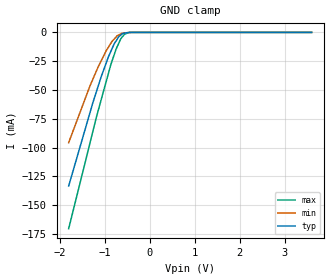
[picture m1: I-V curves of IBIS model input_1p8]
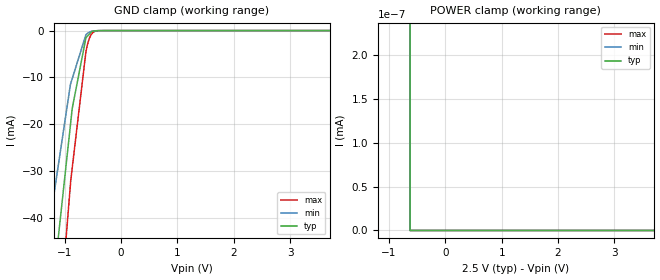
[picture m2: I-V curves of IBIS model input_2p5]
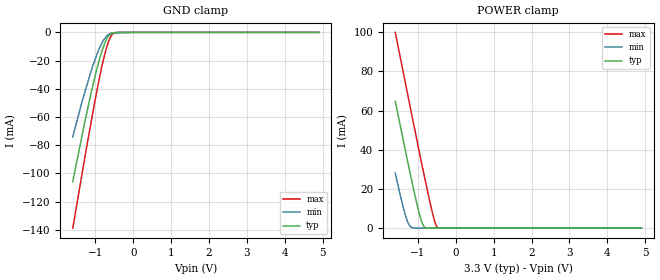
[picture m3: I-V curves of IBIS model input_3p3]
| Texas Instruments Incorporated
| 2N7001T-Q1 Single-Bit Dual-Supply Buffered Voltage Signal Converter
[IBIS Ver]   4.1
[File name]   2n7001t-q1.ibs
[File Rev]   1.0
[Date]   05/25/2018
[Source]
| Texas Instruments Incorporated.
| Analog-eLab Design Center, HPA
| 12500 TI Blvd
| Dallas, TX -75243
[Notes]   Revision History:
| Rev 1.0: 05/25/2018
| - Initial version of the model.
| - Model generated from simulations in SPECTRE.
| - C_comp although listed in numerical order of value are
|   obtained from varying PVT conditions. For PVT conditions for
|   each specific value refer the buffer description under
|   respective [Model]. IBIS model user is responsible for using
|   appropriate C_comp to simulate for Signal Integrity.
| - Model names with a trailing _1p8 contain the model for 1.8V operation.
|   Model names with a trailing _2p5 contain the model for 2.5V operation.
|   Model names with a trailing _3p3 contain the model for 3.3V operation.
[Disclaimer]
| This model is designed as an aid for customers of Texas Instruments.
| TI and its licensors and suppliers make no warranties, either expressed
| or implied, with respect to this  model, including the warranties of
| merchantability or fitness for a particular purpose. The model is
| provided solely on an "as is" basis. The entire risk as to its quality
| and performance is with the customer.
| This model is subject to change without notice. Texas Instruments
| Incorporated is not responsible for updating this model.
[Copyright]
(C) Copyright 2018 Texas Instruments Incorporated.All rights reserved.
|  Component 2N7001TQDCKRQ1 5-pin SC70 - DCK Package
|  Part # 2N7001TQDCKRQ1
[Component]   2N7001TQDCKRQ1
[Manufacturer]   TI
[Package]   |5 SC70 - DCK Package
|   typ   min   max
R_pkg   0.05   0.04   0.06
L_pkg   1.0nH   0.8nH   1.2nH
C_pkg   0.2pF   0.16pF   0.24pF
[Pin]   signal_name   model_name   R_pin   L_pin   C_pin
1   B   output   NA   NA   NA
2   VCCB   power   NA   NA   NA
3   GND   gnd   NA   NA   NA
4   A   input   NA   NA   NA
5   VCCA   power   NA   NA   NA
|   Model Selectors
[Model Selector]   output
output_1p8   1.8V   Digital Output
output_2p5   2.5V   Digital Output
output_3p3   3.3V   Digital Output
[Model Selector]   input
input_1p8   1.8V   Digital Input
input_2p5   2.5V   Digital Input
input_3p3   3.3V   Digital Input
| Models and submodels in the file (6): input_1p8 (Input), input_2p5 (Input), input_3p3 (Input), output_1p8 (Output), output_2p5 (Output), output_3p3 (Output)
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|   input_1p8 Model
[Model]   input_1p8
Model_type   Input
Vinl = 0.63
Vinh = 1.17
|   typ   min   max
C_comp   0.4871pF   0.3678pF   0.7475pF
|  Where Nom  PVT is Nominal Process,   1.8V,  27C
|   Fast PVT is Strong Process,   1.95V, -40C
|   Slow PVT is Weak Process,   1.65V, 130C
[Model spec]
|subparameter
Vinl   0.63   0.578   0.683
Vinh   1.17   1.073   1.268
[Voltage Range]   1.8   1.65   1.95
|Junction Temperature
[Temperature Range]   27   130   -40
[Power Clamp Reference]   1.8   1.65   1.95
[GND Clamp Reference]   0   0   0
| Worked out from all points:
|   GND clamp passes 1 mA (typ) near -0.60 V on its own axis
[GND Clamp]
|   Voltage   I(typ)   I(min)   I(max)
-1.8V     -133.4mA   -95.76mA   -170.5mA
-1.329V   -70.02mA   -46.69mA   -96.49mA
-1.176V   -50.62mA   -32.84mA   -72.54mA
-1.076V   -38.35mA   -24.46mA   -58.21mA
-918.3mV  -21.41mA   -12.94mA   -35.86mA
-862mV    -16.42mA   -9.398mA   -27.85mA
-743.7mV  -7.233mA   -3.863mA   -14.32mA
-686.9mV  -3.715mA   -2.245mA   -9.459mA
-640.9mV  -2.343mA   -1.317mA   -5.512mA
-555.4mV  -622.7uA   -479.8uA   -1.411mA
-372.2mV  -3.465uA   -6.978uA   -8.321uA
3.6V      0A         0A         0A
[POWER Clamp]
|   Voltage   I(typ)   I(min)   I(max)
-1.8V     0A         0A         0A
0V        0A         0A         0A
3.6V      0A         0A         0A
|   input_2p5 Model
[Model]   input_2p5
Model_type   Input
Vinl = 0.7
Vinh = 1.6
|   typ   min   max
C_comp   0.6021pF   0.407pF   0.8544pF
|  Where Nom  PVT is Nominal Process,   2.5V,  27C
|   Fast PVT is Strong Process,   2.7V, -40C
|   Slow PVT is Weak Process,   2.3V, 130C
[Voltage Range]   2.5   2.3   2.7
|Junction Temperature
[Temperature Range]   27   130   -40
[Power Clamp Reference]   2.5   2.3   2.7
[GND Clamp Reference]   0   0   0
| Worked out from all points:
|   GND clamp passes 1 mA (typ) near -0.58 V on its own axis
|   POWER clamp passes 1 mA (typ) near -1.65 V on its own axis
[GND Clamp]
|   Voltage   I(typ)   I(min)   I(max)
-2.5V     -235.9mA   -175.5mA   -1.819A
-1.353V   -73.9mA    -50.2mA    -99.92mA
-1.273V   -62.98mA   -41.43mA   -88.06mA
-1.222V   -56.03mA   -37.34mA   -80.51mA
-899.7mV  -20.15mA   -11.48mA   -32.82mA
-868.2mV  -16.64mA   -10.27mA   -29.34mA
-625mV    -1.529mA   -877.6uA   -4.494mA
-583.8mV  -1.011mA   -466.9uA   -2.4mA
-560.4mV  -718uA     -339.6uA   -1.561mA
-514.7mV  -165.9uA   -140.6uA   -575.4uA
-409.2mV  -13.07uA   -21.38uA   -29.47uA
5V        0A         0A         0A
[POWER Clamp]
|   Voltage   I(typ)   I(min)   I(max)
-2.5V     74.25mA    46.22mA    99.87mA
-1.342V   32.99uA    19.24uA    58.86uA
-625mV    0A         175pA      120.1pA
-624.9mV  0A         135.8pA    0A
-624.9mV  0A         0A         0A
5V        0A         0A         0A
|   input_3p3 Model
[Model]   input_3p3
Model_type   Input
Vinl = 0.8
Vinh = 2.0
|   typ   min   max
C_comp   0.6977pF   0.4525pF   0.8988pF
|  Where Nom  PVT is Nominal Process,   3.3V,  27C
|   Fast PVT is Strong Process,   3.6V, -40C
|   Slow PVT is Weak Process,   3V, 130C
[Voltage Range]   3.3   3   3.6
|Junction Temperature
[Temperature Range]   27   130   -40
[Power Clamp Reference]   3.3   3   3.6
[GND Clamp Reference]   0   0   0
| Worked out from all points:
|   GND clamp passes 1 mA (typ) near -0.59 V on its own axis
|   POWER clamp passes 1 mA (typ) near -0.85 V on its own axis
[GND Clamp]
|   Voltage   I(typ)   I(min)   I(max)
-1.6V     -105.9mA   -74.14mA   -138.8mA
-1.35V    -72.59mA   -48.77mA   -99.65mA
-1.136V   -45.54mA   -29.18mA   -66.74mA
-988.8mV  -28.67mA   -17.62mA   -44.95mA
-901.4mV  -19.75mA   -11.69mA   -32.98mA
-794.2mV  -10.53mA   -5.719mA   -19.87mA
-752.5mV  -7.4mA     -4.25mA    -15.25mA
-689.1mV  -3.894mA   -2.058mA   -9.213mA
-643mV    -2.231mA   -1.38mA    -5.656mA
-557.6mV  -451.9uA   -410.9uA   -1.476mA
-410.3mV  -28.5uA    -302.4uA   -30.58uA
4.9V      0A         0A         0A
[POWER Clamp]
|   Voltage   I(typ)   I(min)   I(max)
-1.6V     64.7mA     28.13mA    99.87mA
-1.395V   45.43mA    11.06mA    80.11mA
-1.266V   33.38mA    2.902mA    67.67mA
-1.196V   26.99mA    729uA      60.92mA
-1.146V   22.49mA    199.1uA    56.07mA
-1.016V   11.35mA    19.9uA     43.72mA
-910.7mV  3.752mA    17.83uA    33.82mA
-825.1mV  489.7uA    16.16uA    25.87mA
-602.8mV  42.31uA    11.8uA     6.556mA
-530.2mV  37.22uA    10.38uA    1.87mA
-484.4mV  34uA       9.485uA    400uA
4.9V      0A         0A         0A
